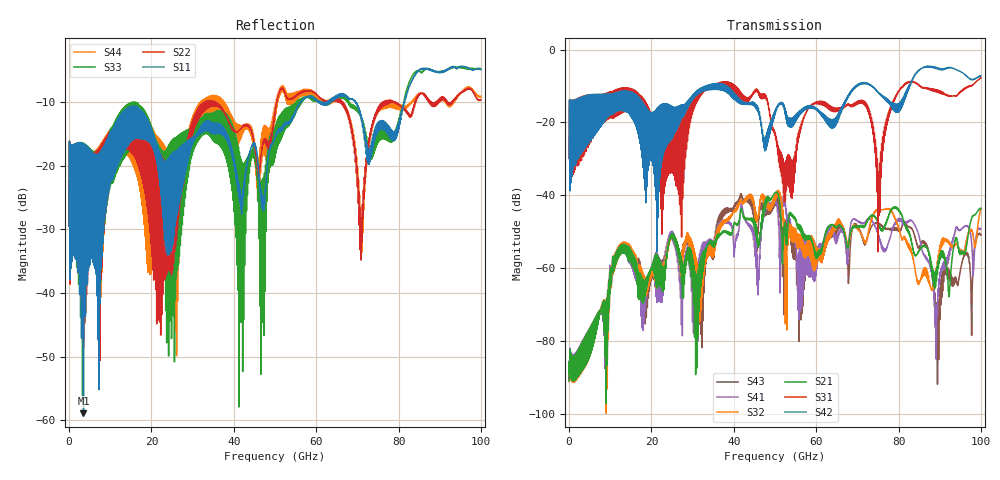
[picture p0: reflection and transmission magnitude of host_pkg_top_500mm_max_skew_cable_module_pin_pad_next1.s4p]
# Hz S RI R 50
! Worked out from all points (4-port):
!   10000 points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, 10 MHz to 100 GHz, reference 50 ohm
!   strongest paths, dB at 10 MHz, 25.01 GHz, 50.01 GHz, 75.01 GHz, 100 GHz:
!     S42: -29.9, -15.8, -16.8, -11.6, -7.2
!     S31: -29.9, -26.4, -23.1, -42.2, -7.7
!     S21: -91.1, -50.6, -39.3, -47.6, -43.8
!     S32: -91.2, -51.3, -39.8, -43.9, -43.8
!     S41: -90.8, -49.9, -41.4, -50.5, -49.4
!     S43: -90.9, -50.4, -40.6, -47.6, -51.0
!   lowest |S11| = -58.9 dB at 3.5 GHz (marker M1), VSWR 1.00, Z = 49.9 + j0.0637 ohm
!   |S11| at or under -10 dB: start of sweep to 56.22 GHz; 61.11 GHz to 62.71 GHz (1.598 GHz wide, 2.58 % of centre); 69.55 GHz to 81.5 GHz (11.95 GHz wide, 15.8 % of centre)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
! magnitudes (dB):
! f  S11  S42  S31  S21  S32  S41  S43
! 10 MHz  -29.5  -29.9  -29.9  -91.1  -91.2  -90.8  -90.9
! 3.5 GHz  -58.9  -26.1  -22.3  -80.1  -80.4  -79.8  -80.2
! 41.63 GHz  -25.6  -14.8  -12.0  -44.3  -41.3  -43.9  -39.6
! 71.55 GHz  -14.3  -9.2  -14.1  -48.5  -52.2  -47.8  -53.2
! 75.16 GHz  -14.1  -11.8  -34.4  -48.0  -43.9  -51.4  -47.8
! 89.39 GHz  -5.3  -5.0  -11.1  -60.7  -58.4  -72.0  -76.0
! 100 GHz  -4.9  -7.2  -7.7  -43.8  -43.8  -49.4  -51.0
